|   Microchip Technology Inc.
|   PolarFire IBIS Model
[IBIS ver]   5.0
[File name]   polarfire_hsio_se.ibs
[File Rev]   2.2
[Date]   Wed Nov 22 2023
[Source] Simulated Models ONLY.
   All data is based on Spice simulation. All performed at Microchip Technology Inc.
[Notes]   This IBIS file is for HSIO single ended standards.
   Please refer to polarfire_hsio_diff.ibs for HSIO differential Standards Configurations,
   and refer to polarfire_gpio_se.ibs and polarfire_gpio_diff.ibs for GPIO Configurations.
   The package parasitics of various package types are given.
   Uncomment the appropriate package before simulations.
   Revision History
   Rev 2.2: 22-Nov-2023
   - Added mixed mode receiver support:
   - Input buffers: LVCMOS12_135_ODT-OFF,LVCMOS12_135_ODT-120,LVCMOS12_135_ODT-240,
   HSTL12_18_ODT-OFF,HSTL12_15_ODT-OFF,HSTL12_135_ODT-OFF,
   HSTL135_18_ODT-OFF,HSTL135_15_ODT-OFF,HSTL15_18_ODT-OFF,
   HSUL12_18_ODT-OFF,HSUL12_18_ODT-60,HSUL12_18_ODT-120,HSUL12_18_ODT-240,
   HSUL12_15_ODT-OFF,HSUL12_15_ODT-60,HSUL12_15_ODT-120,HSUL12_15_ODT-240,
   HSUL12_135_ODT-OFF,HSUL12_135_ODT-60,HSUL12_135_ODT-120,HSUL12_135_ODT-240,
   POD12_18_ODT-OFF,POD12_15_ODT-OFF,POD12_135_ODT-OFF,SSTL135_18_ODT-OFF,
   SSTL135_15_ODT-OFF,SSTL15_18_ODT-OFF
   Rev 2.1: 14-Sep-2022
   - Added MPF050 device with RLC package data in [Package] section
   - Component name change to PolarFire
   - Added LPDDR4 LVSTL11 I/O standard
   - Added RLC package type of FCG784N for MPF300T/TS device
   - Update RLC values of 200T-FCVG484 device package data
[Disclaimer] This information is for board design considerations.
   Simulation based V/I curves contained in this model file are
   considered preliminary until verified against bench
   measurements. Maximum currents may vary from part to part but
   should not exceed maximum I/V curves provided in this model file.
[Copyright]  (c) 2023, Microchip Technology Inc., All Rights Reserved.
| ADDITIONAL NOTES
| Warnings for ISSO Pullup, Pulldown currents being non-zero maybe ignored.
| The naming conventions used in the signal_name/model_name are as follows:
| SLEW-#  - Slew setting,OFF or ON represented by #
| HYST-#  - Hysteresis setting,OFF or ON represented by #
| #mA   - Driver current strength, value represented by #
| #ohm   - Driver impedance mode, value represented by #
| ODT-#   - Series on-die termination, impedance value represented by #
| C1   - Refers to Class-I driver models
| C2   - Refers to Class-II driver models
| #_I   - Refers to input models ,  model name represented by #
| #_O   - Refers to output models , model name represented by #
| IBIS MODEL CHECKLIST
| Microchip Technology Inc. is dedicated to releasing quality IBIS models to customers.
| The following items have been
| verified for this IBIS model before release:
| 1)  Checked IBIS model by the golden parser ibischk5 [Complete]
| 2)  Ensured no errors reported by golden parser
|   for the IBIS model [Complete]
| 3)  Defined Vinl and Vinh for receivers [Complete]
| 4)  Defined Standard Load and Vmeas values for drivers [Complete]
| 5)  Defined overshoots for drivers and receivers [NA]
| 6)  Validated Ramp Values[]
| 7)  Defined V-T Tables for all output drivers [Complete]
| 8)  Validated [Diff Pins] [NA]
| 9)  Verified Package Parasitics [Complete]
| 10) Defined Standard Load Parameters and Specifications
|   for waveforms [Complete]
| 11) Defined and Validate Pin mappings [Complete]
| 12) Verified C_comp_pullup and C_comp_pulldown Values []
| 13) Visually Inspected I-V Curves and V-T Tables  [Complete]
| 14) Presented Typ/Min/Max Values in the correct order for
|   all tables and parameters [Complete]
| 15) Simulated all output models with standard load and
|   switching through Vmeas [Complete]
| 16) Simulated all receiver models  [Complete]
| 17) Validated Models selectors. [NA]
| 18) Visually inspected Spice and IBIS correlation for
|   a) Typical VT Curves [Complete]
|   b) Minimum VT Curves [Complete]
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[Component]   PolarFire
[Manufacturer]   Microchip Technology Inc.
[Package]
|   typ   min   max
|MPF050T/TL/TLS/TS
|R_pkg   0.424   NA   NA   | MPF050T/TL/TLS/TS-FCSG325
|L_pkg   2.847nH   NA   NA   | MPF050T/TL/TLS/TS-FCSG325
|C_pkg   1.075pF   NA   NA   | MPF050T/TL/TLS/TS-FCSG325
|R_pkg   0.726   NA   NA   | MPF050T/TL/TLS/TS-FCVG484
|L_pkg   5.270nH   NA   NA   | MPF050T/TL/TLS/TS-FCVG484
|C_pkg   1.827pF   NA   NA   | MPF050T/TL/TLS/TS-FCVG484
|MPF100T/TL/TLS/TS
|R_pkg   0.300925   NA   NA   | MPF100T/TL/TLS/TS-FCSG325
|L_pkg   2.47653nH   NA   NA   | MPF100T/TL/TLS/TS-FCSG325
|C_pkg   1.00755pF   NA   NA   | MPF100T/TL/TLS/TS-FCSG325
|R_pkg   0.873007   NA   NA   | MPF100T/TL/TLS/TS-FCG484
|L_pkg   5.7244nH   NA   NA   | MPF100T/TL/TLS/TS-FCG484
|C_pkg   2.04208pF   NA   NA   | MPF100T/TL/TLS/TS-FCG484
|R_pkg   0.61   NA   NA   | MPF100T/TL/TLS/TS-FCVG484
|L_pkg   4.49536nH   NA   NA   | MPF100T/TL/TLS/TS-FCVG484
|C_pkg   1.77743pF   NA   NA   | MPF100T/TL/TLS/TS-FCVG484
|MPF200T/TL/TLS/TS
|R_pkg   0.570552   NA   NA   | MPF200T/TL/TLS/TS-FCSG325
|L_pkg   4.57321nH   NA   NA   | MPF200T/TL/TLS/TS-FCSG325
|C_pkg   1.39793pF   NA   NA   | MPF200T/TL/TLS/TS-FCSG325
|R_pkg   0.813737   NA   NA   | MPF200T/TL/TLS/TS-FCG484
|L_pkg   5.39433nH   NA   NA   | MPF200T/TL/TLS/TS-FCG484
|C_pkg   1.90867pF   NA   NA   | MPF200T/TL/TLS/TS-FCG484
|R_pkg   0.592554   NA   NA   | MPF200T/TL/TLS/TS-FCVG484
|L_pkg   4.00867nH   NA   NA   | MPF200T/TL/TLS/TS-FCVG484
|C_pkg   1.56354pF   NA   NA   | MPF200T/TL/TLS/TS-FCVG484
|R_pkg   0.39999   NA   NA   | MPF200T/TL/TLS/TS-FCSG536
|L_pkg   3.20603nH   NA   NA   | MPF200T/TL/TLS/TS-FCSG536
|C_pkg   1.22995pF   NA   NA   | MPF200T/TL/TLS/TS-FCSG536
|R_pkg   1.32073   NA   NA   | MPF200T/TL/TLS/TS-FCG784
|L_pkg   8.15293nH   NA   NA   | MPF200T/TL/TLS/TS-FCG784
|C_pkg   2.72193pF   NA   NA   | MPF200T/TL/TLS/TS-FCG784
|MPF300T/TL/TLS/TS
|R_pkg   0.713491   NA   NA   | MPF300T/TL/TLS/TS-FCG484
|L_pkg   4.77635nH   NA   NA   | MPF300T/TL/TLS/TS-FCG484
|C_pkg   1.82577pF   NA   NA   | MPF300T/TL/TLS/TS-FCG484
|R_pkg   0.493927   NA   NA   | MPF300T/TL/TLS/TS-FCVG484
|L_pkg   3.29806nH   NA   NA   | MPF300T/TL/TLS/TS-FCVG484
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R_pkg   1.65645   NA   NA   | MPF300T/TL/TLS/TS-FCG1152
L_pkg   9.92288nH   NA   NA   | MPF300T/TL/TLS/TS-FCG1152
C_pkg   3.06321pF   NA   NA   | MPF300T/TL/TLS/TS-FCG1152
|MPF500T/TL/TLS/TS
|R_pkg   0.914871   NA   NA   | MPF500T/TL/TLS/TS-FCG784
|L_pkg   5.88658nH   NA   NA   | MPF500T/TL/TLS/TS-FCG784
|C_pkg   2.0993pF   NA   NA   | MPF500T/TL/TLS/TS-FCG784
|R_pkg   1.46382   NA   NA   | MPF500T/TL/TLS/TS-FCG1152
|L_pkg   9.31721nH   NA   NA   | MPF500T/TL/TLS/TS-FCG1152
|C_pkg   2.98723pF   NA   NA   | MPF500T/TL/TLS/TS-FCG1152
| End Header
| The PIN numbers given below are examples. They do not correspond to
| device pin numbers.
[Pin]   signal_name   model_name   R_pin   L_pin   C_pin
1   LVCMOS18_8mA_SLEW-OFF_O   LVCMOS18_8mA_SLEW-OFF_HSIO_O
2   LVCMOS18_2mA_SLEW-OFF_O   LVCMOS18_2mA_SLEW-OFF_HSIO_O
3   LVCMOS18_4mA_SLEW-OFF_O   LVCMOS18_4mA_SLEW-OFF_HSIO_O
4   LVCMOS18_6mA_SLEW-OFF_O   LVCMOS18_6mA_SLEW-OFF_HSIO_O
5   LVCMOS18_10mA_SLEW-OFF_O   LVCMOS18_10mA_SLEW-OFF_HSIO_O
6   LVCMOS18_12mA_SLEW-OFF_O   LVCMOS18_12mA_SLEW-OFF_HSIO_O
7   LVCMOS15_8mA_SLEW-OFF_O   LVCMOS15_8mA_SLEW-OFF_HSIO_O
8   LVCMOS15_2mA_SLEW-OFF_O   LVCMOS15_2mA_SLEW-OFF_HSIO_O
9   LVCMOS15_4mA_SLEW-OFF_O   LVCMOS15_4mA_SLEW-OFF_HSIO_O
10   LVCMOS15_6mA_SLEW-OFF_O   LVCMOS15_6mA_SLEW-OFF_HSIO_O
11   LVCMOS15_10mA_SLEW-OFF_O   LVCMOS15_10mA_SLEW-OFF_HSIO_O
12   LVCMOS12_8mA_SLEW-OFF_O   LVCMOS12_8mA_SLEW-OFF_HSIO_O
13   LVCMOS12_2mA_SLEW-OFF_O   LVCMOS12_2mA_SLEW-OFF_HSIO_O
14   LVCMOS12_4mA_SLEW-OFF_O   LVCMOS12_4mA_SLEW-OFF_HSIO_O
15   LVCMOS12_6mA_SLEW-OFF_O   LVCMOS12_6mA_SLEW-OFF_HSIO_O
16   LVCMOS12_10mA_SLEW-OFF_O   LVCMOS12_10mA_SLEW-OFF_HSIO_O
17   SSTL18_C1_60ohm_SLEW-OFF_O   SSTL18_C1_60ohm_SLEW-OFF_HSIO_O
18   SSTL18_C1_80ohm_SLEW-OFF_O   SSTL18_C1_80ohm_SLEW-OFF_HSIO_O
19   SSTL18_C1_48ohm_SLEW-OFF_O   SSTL18_C1_48ohm_SLEW-OFF_HSIO_O
20   SSTL18_C1_40ohm_SLEW-OFF_O   SSTL18_C1_40ohm_SLEW-OFF_HSIO_O
21   SSTL18_C2_40ohm_SLEW-OFF_O   SSTL18_C2_40ohm_SLEW-OFF_HSIO_O
22   SSTL18_C2_48ohm_SLEW-OFF_O   SSTL18_C2_48ohm_SLEW-OFF_HSIO_O
23   SSTL18_C2_34ohm_SLEW-OFF_O   SSTL18_C2_34ohm_SLEW-OFF_HSIO_O
24   SSTL18_C2_30ohm_SLEW-OFF_O   SSTL18_C2_30ohm_SLEW-OFF_HSIO_O
25   SSTL15_C1_40ohm_SLEW-OFF_O   SSTL15_C1_40ohm_SLEW-OFF_HSIO_O
26   SSTL15_C1_48ohm_SLEW-OFF_O   SSTL15_C1_48ohm_SLEW-OFF_HSIO_O
27   SSTL15_C2_34ohm_SLEW-OFF_O   SSTL15_C2_34ohm_SLEW-OFF_HSIO_O
28   SSTL15_C2_30ohm_SLEW-OFF_O   SSTL15_C2_30ohm_SLEW-OFF_HSIO_O
29   SSTL15_C2_27ohm_SLEW-OFF_O   SSTL15_C2_27ohm_SLEW-OFF_HSIO_O
30   SSTL135_C1_40ohm_SLEW-OFF_O   SSTL135_C1_40ohm_SLEW-OFF_HSIO_O
31   SSTL135_C1_48ohm_SLEW-OFF_O   SSTL135_C1_48ohm_SLEW-OFF_HSIO_O
32   SSTL135_C2_34ohm_SLEW-OFF_O   SSTL135_C2_34ohm_SLEW-OFF_HSIO_O
33   SSTL135_C2_30ohm_SLEW-OFF_O   SSTL135_C2_30ohm_SLEW-OFF_HSIO_O
34   SSTL135_C2_27ohm_SLEW-OFF_O   SSTL135_C2_27ohm_SLEW-OFF_HSIO_O
35   HSUL18_C1_55ohm_SLEW-OFF_O   HSUL18_C1_55ohm_SLEW-OFF_HSIO_O
36   HSUL18_C1_60ohm_SLEW-OFF_O   HSUL18_C1_60ohm_SLEW-OFF_HSIO_O
37   HSUL18_C1_40ohm_SLEW-OFF_O   HSUL18_C1_40ohm_SLEW-OFF_HSIO_O
38   HSUL18_C1_34ohm_SLEW-OFF_O   HSUL18_C1_34ohm_SLEW-OFF_HSIO_O
39   HSUL18_C2_25ohm_SLEW-OFF_O   HSUL18_C2_25ohm_SLEW-OFF_HSIO_O
40   HSUL18_C2_30ohm_SLEW-OFF_O   HSUL18_C2_30ohm_SLEW-OFF_HSIO_O
41   HSUL18_C2_27ohm_SLEW-OFF_O   HSUL18_C2_27ohm_SLEW-OFF_HSIO_O
42   HSUL18_C2_22ohm_SLEW-OFF_O   HSUL18_C2_22ohm_SLEW-OFF_HSIO_O
43   HSTL15_C1_50ohm_SLEW-OFF_O   HSTL15_C1_50ohm_SLEW-OFF_HSIO_O
44   HSTL15_C1_60ohm_SLEW-OFF_O   HSTL15_C1_60ohm_SLEW-OFF_HSIO_O
45   HSTL15_C1_40ohm_SLEW-OFF_O   HSTL15_C1_40ohm_SLEW-OFF_HSIO_O
46   HSTL15_C1_34ohm_SLEW-OFF_O   HSTL15_C1_34ohm_SLEW-OFF_HSIO_O
47   HSTL15_C2_25ohm_SLEW-OFF_O   HSTL15_C2_25ohm_SLEW-OFF_HSIO_O
48   HSTL15_C2_30ohm_SLEW-OFF_O   HSTL15_C2_30ohm_SLEW-OFF_HSIO_O
49   HSTL15_C2_27ohm_SLEW-OFF_O   HSTL15_C2_27ohm_SLEW-OFF_HSIO_O
50   HSTL15_C2_22ohm_SLEW-OFF_O   HSTL15_C2_22ohm_SLEW-OFF_HSIO_O
51   HSTL135_C1_50ohm_SLEW-OFF_O   HSTL135_C1_50ohm_SLEW-OFF_HSIO_O
52   HSTL135_C1_60ohm_SLEW-OFF_O   HSTL135_C1_60ohm_SLEW-OFF_HSIO_O
53   HSTL135_C1_40ohm_SLEW-OFF_O   HSTL135_C1_40ohm_SLEW-OFF_HSIO_O
54   HSTL135_C1_34ohm_SLEW-OFF_O   HSTL135_C1_34ohm_SLEW-OFF_HSIO_O
55   HSTL135_C2_25ohm_SLEW-OFF_O   HSTL135_C2_25ohm_SLEW-OFF_HSIO_O
56   HSTL135_C2_30ohm_SLEW-OFF_O   HSTL135_C2_30ohm_SLEW-OFF_HSIO_O
57   HSTL135_C2_27ohm_SLEW-OFF_O   HSTL135_C2_27ohm_SLEW-OFF_HSIO_O
58   HSTL135_C2_22ohm_SLEW-OFF_O   HSTL135_C2_22ohm_SLEW-OFF_HSIO_O
59   HSUL12_40ohm_SLEW-OFF_O   HSUL12_40ohm_SLEW-OFF_HSIO_O
60   HSUL12_120ohm_SLEW-OFF_O   HSUL12_120ohm_SLEW-OFF_HSIO_O
61   HSUL12_80ohm_SLEW-OFF_O   HSUL12_80ohm_SLEW-OFF_HSIO_O
62   HSUL12_60ohm_SLEW-OFF_O   HSUL12_60ohm_SLEW-OFF_HSIO_O
63   HSUL12_48ohm_SLEW-OFF_O   HSUL12_48ohm_SLEW-OFF_HSIO_O
64   HSUL12_34ohm_SLEW-OFF_O   HSUL12_34ohm_SLEW-OFF_HSIO_O
65   POD12_C1_48ohm_SLEW-OFF_O   POD12_C1_48ohm_SLEW-OFF_HSIO_O
66   POD12_C1_60ohm_SLEW-OFF_O   POD12_C1_60ohm_SLEW-OFF_HSIO_O
67   POD12_C1_40ohm_SLEW-OFF_O   POD12_C1_40ohm_SLEW-OFF_HSIO_O
68   POD12_C2_34ohm_SLEW-OFF_O   POD12_C2_34ohm_SLEW-OFF_HSIO_O
69   POD12_C2_30ohm_SLEW-OFF_O   POD12_C2_30ohm_SLEW-OFF_HSIO_O
70   POD12_C2_27ohm_SLEW-OFF_O   POD12_C2_27ohm_SLEW-OFF_HSIO_O
71   HSTL12_C1_50ohm_SLEW-OFF_O   HSTL12_C1_50ohm_SLEW-OFF_HSIO_O
72   HSTL12_C2_25ohm_SLEW-OFF_O   HSTL12_C2_25ohm_SLEW-OFF_HSIO_O
73   LVCMOS18_ODT-OFF_HYST-ON_I   LVCMOS18_ODT-OFF_HYST-ON_HSIO_I
74   LVCMOS18_ODT-OFF_HYST-OFF_I   LVCMOS18_ODT-OFF_HYST-OFF_HSIO_I
75   LVCMOS18_ODT-120_HYST-ON_I   LVCMOS18_ODT-120_HYST-ON_HSIO_I
76   LVCMOS18_ODT-240_HYST-ON_I   LVCMOS18_ODT-240_HYST-ON_HSIO_I
77   LVCMOS18_ODT-120_HYST-OFF_I   LVCMOS18_ODT-120_HYST-OFF_HSIO_I
78   LVCMOS18_ODT-240_HYST-OFF_I   LVCMOS18_ODT-240_HYST-OFF_HSIO_I
79   LVCMOS15_18_ODT-OFF_HYST-ON_I   LVCMOS15_18_ODT-OFF_HYST-ON_HSIO_I
80   LVCMOS15_18_ODT-OFF_HYST-OFF_I   LVCMOS15_18_ODT-OFF_HYST-OFF_HSIO_I
81   LVCMOS15_18_ODT-120_HYST-ON_I   LVCMOS15_18_ODT-120_HYST-ON_HSIO_I
82   LVCMOS15_18_ODT-240_HYST-ON_I   LVCMOS15_18_ODT-240_HYST-ON_HSIO_I
83   LVCMOS15_18_ODT-120_HYST-OFF_I   LVCMOS15_18_ODT-120_HYST-OFF_HSIO_I
84   LVCMOS15_18_ODT-240_HYST-OFF_I   LVCMOS15_18_ODT-240_HYST-OFF_HSIO_I
85   LVCMOS15_ODT-OFF_HYST-ON_I   LVCMOS15_ODT-OFF_HYST-ON_HSIO_I
86   LVCMOS15_ODT-OFF_HYST-OFF_I   LVCMOS15_ODT-OFF_HYST-OFF_HSIO_I
87   LVCMOS15_ODT-120_HYST-ON_I   LVCMOS15_ODT-120_HYST-ON_HSIO_I
88   LVCMOS15_ODT-240_HYST-ON_I   LVCMOS15_ODT-240_HYST-ON_HSIO_I
89   LVCMOS15_ODT-120_HYST-OFF_I   LVCMOS15_ODT-120_HYST-OFF_HSIO_I
90   LVCMOS15_ODT-240_HYST-OFF_I   LVCMOS15_ODT-240_HYST-OFF_HSIO_I
91   LVCMOS12_18_ODT-OFF_HYST-OFF_I   LVCMOS12_18_ODT-OFF_HYST-OFF_HSIO_I
92   LVCMOS12_15_ODT-OFF_HYST-OFF_I   LVCMOS12_15_ODT-OFF_HYST-OFF_HSIO_I
93   LVCMOS12_18_ODT-120_HYST-OFF_I   LVCMOS12_18_ODT-120_HYST-OFF_HSIO_I
94   LVCMOS12_15_ODT-120_HYST-OFF_I   LVCMOS12_15_ODT-120_HYST-OFF_HSIO_I
95   LVCMOS12_18_ODT-240_HYST-OFF_I   LVCMOS12_18_ODT-240_HYST-OFF_HSIO_I
96   LVCMOS12_15_ODT-240_HYST-OFF_I   LVCMOS12_15_ODT-240_HYST-OFF_HSIO_I
97   LVCMOS12_ODT-OFF_HYST-OFF_I   LVCMOS12_ODT-OFF_HYST-OFF_HSIO_I
98   LVCMOS12_ODT-120_HYST-OFF_I   LVCMOS12_ODT-120_HYST-OFF_HSIO_I
99   LVCMOS12_ODT-240_HYST-OFF_I   LVCMOS12_ODT-240_HYST-OFF_HSIO_I
100   SSTL18_ODT-OFF_HYST-OFF_I   SSTL18_ODT-OFF_HYST-OFF_HSIO_I
101   SSTL18_ODT-50_HYST-OFF_I   SSTL18_ODT-50_HYST-OFF_HSIO_I
102   SSTL18_ODT-150_HYST-OFF_I   SSTL18_ODT-150_HYST-OFF_HSIO_I
103   SSTL18_ODT-75_HYST-OFF_I   SSTL18_ODT-75_HYST-OFF_HSIO_I
104   SSTL15_ODT-OFF_HYST-OFF_I   SSTL15_ODT-OFF_HYST-OFF_HSIO_I
105   SSTL15_ODT-60_HYST-OFF_I   SSTL15_ODT-60_HYST-OFF_HSIO_I
106   SSTL15_ODT-120_HYST-OFF_I   SSTL15_ODT-120_HYST-OFF_HSIO_I
107   SSTL15_ODT-40_HYST-OFF_I   SSTL15_ODT-40_HYST-OFF_HSIO_I
108   SSTL15_ODT-30_HYST-OFF_I   SSTL15_ODT-30_HYST-OFF_HSIO_I
109   SSTL15_ODT-20_HYST-OFF_I   SSTL15_ODT-20_HYST-OFF_HSIO_I
110   SSTL135_ODT-OFF_HYST-OFF_I   SSTL135_ODT-OFF_HYST-OFF_HSIO_I
111   SSTL135_ODT-60_HYST-OFF_I   SSTL135_ODT-60_HYST-OFF_HSIO_I
112   SSTL135_ODT-120_HYST-OFF_I   SSTL135_ODT-120_HYST-OFF_HSIO_I
113   SSTL135_ODT-40_HYST-OFF_I   SSTL135_ODT-40_HYST-OFF_HSIO_I
114   SSTL135_ODT-30_HYST-OFF_I   SSTL135_ODT-30_HYST-OFF_HSIO_I
115   SSTL135_ODT-20_HYST-OFF_I   SSTL135_ODT-20_HYST-OFF_HSIO_I
116   HSUL18_ODT-OFF_HYST-OFF_I   HSUL18_ODT-OFF_HYST-OFF_HSIO_I
117   HSUL18_ODT-50_HYST-OFF_I   HSUL18_ODT-50_HYST-OFF_HSIO_I
118   HSTL15_ODT-OFF_HYST-OFF_I   HSTL15_ODT-OFF_HYST-OFF_HSIO_I
119   HSTL15_ODT-50_HYST-OFF_I   HSTL15_ODT-50_HYST-OFF_HSIO_I
120   HSTL135_ODT-OFF_HYST-OFF_I   HSTL135_ODT-OFF_HYST-OFF_HSIO_I
121   HSTL135_ODT-50_HYST-OFF_I   HSTL135_ODT-50_HYST-OFF_HSIO_I
122   HSUL12_ODT-OFF_HYST-OFF_I   HSUL12_ODT-OFF_HYST-OFF_HSIO_I
123   HSUL12_ODT-60_HYST-OFF_I   HSUL12_ODT-60_HYST-OFF_HSIO_I
124   HSUL12_ODT-240_HYST-OFF_I   HSUL12_ODT-240_HYST-OFF_HSIO_I
125   HSUL12_ODT-120_HYST-OFF_I   HSUL12_ODT-120_HYST-OFF_HSIO_I
126   POD12_ODT-OFF_HYST-OFF_I   POD12_ODT-OFF_HYST-OFF_HSIO_I
127   POD12_ODT-60_HYST-OFF_I   POD12_ODT-60_HYST-OFF_HSIO_I
128   POD12_ODT-240_HYST-OFF_I   POD12_ODT-240_HYST-OFF_HSIO_I
129   POD12_ODT-120_HYST-OFF_I   POD12_ODT-120_HYST-OFF_HSIO_I
130   POD12_ODT-80_HYST-OFF_I   POD12_ODT-80_HYST-OFF_HSIO_I
131   POD12_ODT-48_HYST-OFF_I   POD12_ODT-48_HYST-OFF_HSIO_I
132   POD12_ODT-40_HYST-OFF_I   POD12_ODT-40_HYST-OFF_HSIO_I
133   POD12_ODT-34_HYST-OFF_I   POD12_ODT-34_HYST-OFF_HSIO_I
134   HSTL12_ODT-OFF_HYST-OFF_I   HSTL12_ODT-OFF_HYST-OFF_HSIO_I
135   HSTL12_ODT-50_HYST-OFF_I   HSTL12_ODT-50_HYST-OFF_HSIO_I
136   LVSTL11_C1_40ohm_SLEW-OFF_O   LVSTL11_C1_40ohm_SLEW-OFF_HSIO_O
137   LVSTL11_C1_120ohm_SLEW-OFF_O   LVSTL11_C1_120ohm_SLEW-OFF_HSIO_O
138   LVSTL11_C1_80ohm_SLEW-OFF_O   LVSTL11_C1_80ohm_SLEW-OFF_HSIO_O
139   LVSTL11_C1_60ohm_SLEW-OFF_O   LVSTL11_C1_60ohm_SLEW-OFF_HSIO_O
140   LVSTL11_C1_48ohm_SLEW-OFF_O   LVSTL11_C1_48ohm_SLEW-OFF_HSIO_O
141   LVSTL11_C1_34ohm_SLEW-OFF_O   LVSTL11_C1_34ohm_SLEW-OFF_HSIO_O
142   LVSTL11_ODT-OFF_HYST-OFF_I   LVSTL11_ODT-OFF_HYST-OFF_HSIO_I
143   LVSTL11_ODT-60_HYST-OFF_I   LVSTL11_ODT-60_HYST-OFF_HSIO_I
144   LVSTL11_ODT-120_HYST-OFF_I   LVSTL11_ODT-120_HYST-OFF_HSIO_I
145   LVSTL11_ODT-80_HYST-OFF_I   LVSTL11_ODT-80_HYST-OFF_HSIO_I
146   LVSTL11_ODT-48_HYST-OFF_I   LVSTL11_ODT-48_HYST-OFF_HSIO_I
147   LVSTL11_ODT-40_HYST-OFF_I   LVSTL11_ODT-40_HYST-OFF_HSIO_I
148   LVCMOS12_135_ODT-OFF_HYST-OFF_I   LVCMOS12_135_ODT-OFF_HYST-OFF_HSIO_I
149   LVCMOS12_135_ODT-120_HYST-OFF_I   LVCMOS12_135_ODT-120_HYST-OFF_HSIO_I
150   LVCMOS12_135_ODT-240_HYST-OFF_I   LVCMOS12_135_ODT-240_HYST-OFF_HSIO_I
151   HSTL12_18_ODT-OFF_HYST-OFF_I   HSTL12_18_ODT-OFF_HYST-OFF_HSIO_I
152   HSTL12_15_ODT-OFF_HYST-OFF_I   HSTL12_15_ODT-OFF_HYST-OFF_HSIO_I
153   HSTL12_135_ODT-OFF_HYST-OFF_I   HSTL12_135_ODT-OFF_HYST-OFF_HSIO_I
154   HSTL135_18_ODT-OFF_HYST-OFF_I   HSTL135_18_ODT-OFF_HYST-OFF_HSIO_I
155   HSTL135_15_ODT-OFF_HYST-OFF_I   HSTL135_15_ODT-OFF_HYST-OFF_HSIO_I
156   HSTL15_18_ODT-OFF_HYST-OFF_I   HSTL15_18_ODT-OFF_HYST-OFF_HSIO_I
157   HSUL12_18_ODT-OFF_HYST-OFF_I   HSUL12_18_ODT-OFF_HYST-OFF_HSIO_I
158   HSUL12_15_ODT-OFF_HYST-OFF_I   HSUL12_15_ODT-OFF_HYST-OFF_HSIO_I
159   HSUL12_135_ODT-OFF_HYST-OFF_I   HSUL12_135_ODT-OFF_HYST-OFF_HSIO_I
160   HSUL12_18_ODT-60_HYST-OFF_I   HSUL12_18_ODT-60_HYST-OFF_HSIO_I
161   HSUL12_15_ODT-60_HYST-OFF_I   HSUL12_15_ODT-60_HYST-OFF_HSIO_I
162   HSUL12_135_ODT-60_HYST-OFF_I   HSUL12_135_ODT-60_HYST-OFF_HSIO_I
163   HSUL12_18_ODT-240_HYST-OFF_I   HSUL12_18_ODT-240_HYST-OFF_HSIO_I
164   HSUL12_15_ODT-240_HYST-OFF_I   HSUL12_15_ODT-240_HYST-OFF_HSIO_I
165   HSUL12_135_ODT-240_HYST-OFF_I   HSUL12_135_ODT-240_HYST-OFF_HSIO_I
166   HSUL12_18_ODT-120_HYST-OFF_I   HSUL12_18_ODT-120_HYST-OFF_HSIO_I
167   HSUL12_15_ODT-120_HYST-OFF_I   HSUL12_15_ODT-120_HYST-OFF_HSIO_I
168   HSUL12_135_ODT-120_HYST-OFF_I   HSUL12_135_ODT-120_HYST-OFF_HSIO_I
169   POD12_18_ODT-OFF_HYST-OFF_I   POD12_18_ODT-OFF_HYST-OFF_HSIO_I
170   POD12_15_ODT-OFF_HYST-OFF_I   POD12_15_ODT-OFF_HYST-OFF_HSIO_I
171   POD12_135_ODT-OFF_HYST-OFF_I   POD12_135_ODT-OFF_HYST-OFF_HSIO_I
172   SSTL135_18_ODT-OFF_HYST-OFF_I   SSTL135_18_ODT-OFF_HYST-OFF_HSIO_I
173   SSTL135_15_ODT-OFF_HYST-OFF_I   SSTL135_15_ODT-OFF_HYST-OFF_HSIO_I
174   SSTL15_18_ODT-OFF_HYST-OFF_I   SSTL15_18_ODT-OFF_HYST-OFF_HSIO_I
175   VDDI   POWER
176   VSS   GND
[Pin Mapping]   pulldown_ref   pullup_ref   gnd_clamp_ref   power_clamp_ref   ext_ref
1   VSS   VDDI   VSS   VDDI
2   VSS   VDDI   VSS   VDDI
3   VSS   VDDI   VSS   VDDI
4   VSS   VDDI   VSS   VDDI
5   VSS   VDDI   VSS   VDDI
6   VSS   VDDI   VSS   VDDI
7   VSS   VDDI   VSS   VDDI
8   VSS   VDDI   VSS   VDDI
9   VSS   VDDI   VSS   VDDI
10   VSS   VDDI   VSS   VDDI
11   VSS   VDDI   VSS   VDDI
12   VSS   VDDI   VSS   VDDI
13   VSS   VDDI   VSS   VDDI
14   VSS   VDDI   VSS   VDDI
15   VSS   VDDI   VSS   VDDI
16   VSS   VDDI   VSS   VDDI
17   VSS   VDDI   VSS   VDDI
18   VSS   VDDI   VSS   VDDI
19   VSS   VDDI   VSS   VDDI
20   VSS   VDDI   VSS   VDDI
21   VSS   VDDI   VSS   VDDI
22   VSS   VDDI   VSS   VDDI
23   VSS   VDDI   VSS   VDDI
24   VSS   VDDI   VSS   VDDI
25   VSS   VDDI   VSS   VDDI
26   VSS   VDDI   VSS   VDDI
27   VSS   VDDI   VSS   VDDI
28   VSS   VDDI   VSS   VDDI
29   VSS   VDDI   VSS   VDDI
30   VSS   VDDI   VSS   VDDI
31   VSS   VDDI   VSS   VDDI
32   VSS   VDDI   VSS   VDDI
33   VSS   VDDI   VSS   VDDI
34   VSS   VDDI   VSS   VDDI
35   VSS   VDDI   VSS   VDDI
36   VSS   VDDI   VSS   VDDI
37   VSS   VDDI   VSS   VDDI
38   VSS   VDDI   VSS   VDDI
39   VSS   VDDI   VSS   VDDI
40   VSS   VDDI   VSS   VDDI
41   VSS   VDDI   VSS   VDDI
42   VSS   VDDI   VSS   VDDI
43   VSS   VDDI   VSS   VDDI
44   VSS   VDDI   VSS   VDDI
45   VSS   VDDI   VSS   VDDI
46   VSS   VDDI   VSS   VDDI
47   VSS   VDDI   VSS   VDDI
48   VSS   VDDI   VSS   VDDI
49   VSS   VDDI   VSS   VDDI
50   VSS   VDDI   VSS   VDDI
51   VSS   VDDI   VSS   VDDI
52   VSS   VDDI   VSS   VDDI
53   VSS   VDDI   VSS   VDDI
54   VSS   VDDI   VSS   VDDI
55   VSS   VDDI   VSS   VDDI
56   VSS   VDDI   VSS   VDDI
57   VSS   VDDI   VSS   VDDI
58   VSS   VDDI   VSS   VDDI
59   VSS   VDDI   VSS   VDDI
60   VSS   VDDI   VSS   VDDI
61   VSS   VDDI   VSS   VDDI
62   VSS   VDDI   VSS   VDDI
63   VSS   VDDI   VSS   VDDI
64   VSS   VDDI   VSS   VDDI
65   VSS   VDDI   VSS   VDDI
66   VSS   VDDI   VSS   VDDI
67   VSS   VDDI   VSS   VDDI
68   VSS   VDDI   VSS   VDDI
69   VSS   VDDI   VSS   VDDI
70   VSS   VDDI   VSS   VDDI
71   VSS   VDDI   VSS   VDDI
72   VSS   VDDI   VSS   VDDI
73   VSS   VDDI   VSS   VDDI
74   VSS   VDDI   VSS   VDDI
75   VSS   VDDI   VSS   VDDI
76   VSS   VDDI   VSS   VDDI
77   VSS   VDDI   VSS   VDDI
78   VSS   VDDI   VSS   VDDI
79   VSS   VDDI   VSS   VDDI
80   VSS   VDDI   VSS   VDDI
81   VSS   VDDI   VSS   VDDI
82   VSS   VDDI   VSS   VDDI
83   VSS   VDDI   VSS   VDDI
84   VSS   VDDI   VSS   VDDI
85   VSS   VDDI   VSS   VDDI
86   VSS   VDDI   VSS   VDDI
87   VSS   VDDI   VSS   VDDI
88   VSS   VDDI   VSS   VDDI
89   VSS   VDDI   VSS   VDDI
90   VSS   VDDI   VSS   VDDI
91   VSS   VDDI   VSS   VDDI
92   VSS   VDDI   VSS   VDDI
93   VSS   VDDI   VSS   VDDI
94   VSS   VDDI   VSS   VDDI
95   VSS   VDDI   VSS   VDDI
96   VSS   VDDI   VSS   VDDI
97   VSS   VDDI   VSS   VDDI
98   VSS   VDDI   VSS   VDDI
99   VSS   VDDI   VSS   VDDI
100   VSS   VDDI   VSS   VDDI
101   VSS   VDDI   VSS   VDDI
102   VSS   VDDI   VSS   VDDI
103   VSS   VDDI   VSS   VDDI
104   VSS   VDDI   VSS   VDDI
105   VSS   VDDI   VSS   VDDI
106   VSS   VDDI   VSS   VDDI
107   VSS   VDDI   VSS   VDDI
108   VSS   VDDI   VSS   VDDI
109   VSS   VDDI   VSS   VDDI
110   VSS   VDDI   VSS   VDDI
111   VSS   VDDI   VSS   VDDI
112   VSS   VDDI   VSS   VDDI
113   VSS   VDDI   VSS   VDDI
114   VSS   VDDI   VSS   VDDI
115   VSS   VDDI   VSS   VDDI
116   VSS   VDDI   VSS   VDDI
117   VSS   VDDI   VSS   VDDI
118   VSS   VDDI   VSS   VDDI
119   VSS   VDDI   VSS   VDDI
120   VSS   VDDI   VSS   VDDI
121   VSS   VDDI   VSS   VDDI
122   VSS   VDDI   VSS   VDDI
123   VSS   VDDI   VSS   VDDI
124   VSS   VDDI   VSS   VDDI
125   VSS   VDDI   VSS   VDDI
126   VSS   VDDI   VSS   VDDI
127   VSS   VDDI   VSS   VDDI
128   VSS   VDDI   VSS   VDDI
129   VSS   VDDI   VSS   VDDI
130   VSS   VDDI   VSS   VDDI
131   VSS   VDDI   VSS   VDDI
132   VSS   VDDI   VSS   VDDI
133   VSS   VDDI   VSS   VDDI
134   VSS   VDDI   VSS   VDDI
135   VSS   VDDI   VSS   VDDI
136   VSS   VDDI   VSS   VDDI
137   VSS   VDDI   VSS   VDDI
138   VSS   VDDI   VSS   VDDI
139   VSS   VDDI   VSS   VDDI
140   VSS   VDDI   VSS   VDDI
141   VSS   VDDI   VSS   VDDI
142   VSS   VDDI   VSS   VDDI
143   VSS   VDDI   VSS   VDDI
144   VSS   VDDI   VSS   VDDI
145   VSS   VDDI   VSS   VDDI
146   VSS   VDDI   VSS   VDDI
147   VSS   VDDI   VSS   VDDI
148   VSS   VDDI   VSS   VDDI
149   VSS   VDDI   VSS   VDDI
150   VSS   VDDI   VSS   VDDI
151   VSS   VDDI   VSS   VDDI
152   VSS   VDDI   VSS   VDDI
153   VSS   VDDI   VSS   VDDI
154   VSS   VDDI   VSS   VDDI
155   VSS   VDDI   VSS   VDDI
156   VSS   VDDI   VSS   VDDI
157   VSS   VDDI   VSS   VDDI
158   VSS   VDDI   VSS   VDDI
159   VSS   VDDI   VSS   VDDI
160   VSS   VDDI   VSS   VDDI
161   VSS   VDDI   VSS   VDDI
162   VSS   VDDI   VSS   VDDI
163   VSS   VDDI   VSS   VDDI
164   VSS   VDDI   VSS   VDDI
165   VSS   VDDI   VSS   VDDI
166   VSS   VDDI   VSS   VDDI
167   VSS   VDDI   VSS   VDDI
168   VSS   VDDI   VSS   VDDI
169   VSS   VDDI   VSS   VDDI
170   VSS   VDDI   VSS   VDDI
171   VSS   VDDI   VSS   VDDI
172   VSS   VDDI   VSS   VDDI
173   VSS   VDDI   VSS   VDDI
174   VSS   VDDI   VSS   VDDI
175   NC   VDDI
176   VSS   NC
| Models and submodels in the file (174): LVCMOS18_8mA_SLEW-OFF_HSIO_O (Output), LVCMOS18_2mA_SLEW-OFF_HSIO_O (Output), LVCMOS18_4mA_SLEW-OFF_HSIO_O (Output), LVCMOS18_6mA_SLEW-OFF_HSIO_O (Output), LVCMOS18_10mA_SLEW-OFF_HSIO_O (Output), LVCMOS18_12mA_SLEW-OFF_HSIO_O (Output), LVCMOS15_8mA_SLEW-OFF_HSIO_O (Output), LVCMOS15_2mA_SLEW-OFF_HSIO_O (Output), LVCMOS15_4mA_SLEW-OFF_HSIO_O (Output), LVCMOS15_6mA_SLEW-OFF_HSIO_O (Output), LVCMOS15_10mA_SLEW-OFF_HSIO_O (Output), LVCMOS12_8mA_SLEW-OFF_HSIO_O (Output), LVCMOS12_2mA_SLEW-OFF_HSIO_O (Output), LVCMOS12_4mA_SLEW-OFF_HSIO_O (Output), LVCMOS12_6mA_SLEW-OFF_HSIO_O (Output), LVCMOS12_10mA_SLEW-OFF_HSIO_O (Output), SSTL18_C1_60ohm_SLEW-OFF_HSIO_O (Output), SSTL18_C1_80ohm_SLEW-OFF_HSIO_O (Output), SSTL18_C1_48ohm_SLEW-OFF_HSIO_O (Output), SSTL18_C1_40ohm_SLEW-OFF_HSIO_O (Output), SSTL18_C2_40ohm_SLEW-OFF_HSIO_O (Output), SSTL18_C2_48ohm_SLEW-OFF_HSIO_O (Output), SSTL18_C2_34ohm_SLEW-OFF_HSIO_O (Output), SSTL18_C2_30ohm_SLEW-OFF_HSIO_O (Output), SSTL15_C1_40ohm_SLEW-OFF_HSIO_O (Output), SSTL15_C1_48ohm_SLEW-OFF_HSIO_O (Output), SSTL15_C2_34ohm_SLEW-OFF_HSIO_O (Output), SSTL15_C2_30ohm_SLEW-OFF_HSIO_O (Output), SSTL15_C2_27ohm_SLEW-OFF_HSIO_O (Output), SSTL135_C1_40ohm_SLEW-OFF_HSIO_O (Output), SSTL135_C1_48ohm_SLEW-OFF_HSIO_O (Output), SSTL135_C2_34ohm_SLEW-OFF_HSIO_O (Output), SSTL135_C2_30ohm_SLEW-OFF_HSIO_O (Output), SSTL135_C2_27ohm_SLEW-OFF_HSIO_O (Output), HSUL18_C1_55ohm_SLEW-OFF_HSIO_O (Output), HSUL18_C1_60ohm_SLEW-OFF_HSIO_O (Output), HSUL18_C1_40ohm_SLEW-OFF_HSIO_O (Output), HSUL18_C1_34ohm_SLEW-OFF_HSIO_O (Output), HSUL18_C2_25ohm_SLEW-OFF_HSIO_O (Output), HSUL18_C2_30ohm_SLEW-OFF_HSIO_O (Output), HSUL18_C2_27ohm_SLEW-OFF_HSIO_O (Output), HSUL18_C2_22ohm_SLEW-OFF_HSIO_O (Output), HSTL15_C1_50ohm_SLEW-OFF_HSIO_O (Output), HSTL15_C1_60ohm_SLEW-OFF_HSIO_O (Output), HSTL15_C1_40ohm_SLEW-OFF_HSIO_O (Output), HSTL15_C1_34ohm_SLEW-OFF_HSIO_O (Output), HSTL15_C2_25ohm_SLEW-OFF_HSIO_O (Output), HSTL15_C2_30ohm_SLEW-OFF_HSIO_O (Output), HSTL15_C2_27ohm_SLEW-OFF_HSIO_O (Output), HSTL15_C2_22ohm_SLEW-OFF_HSIO_O (Output), HSTL135_C1_50ohm_SLEW-OFF_HSIO_O (Output), HSTL135_C1_60ohm_SLEW-OFF_HSIO_O (Output), HSTL135_C1_40ohm_SLEW-OFF_HSIO_O (Output), HSTL135_C1_34ohm_SLEW-OFF_HSIO_O (Output), HSTL135_C2_25ohm_SLEW-OFF_HSIO_O (Output), HSTL135_C2_30ohm_SLEW-OFF_HSIO_O (Output), HSTL135_C2_27ohm_SLEW-OFF_HSIO_O (Output), HSTL135_C2_22ohm_SLEW-OFF_HSIO_O (Output), HSUL12_40ohm_SLEW-OFF_HSIO_O (Output), HSUL12_120ohm_SLEW-OFF_HSIO_O (Output), HSUL12_80ohm_SLEW-OFF_HSIO_O (Output), HSUL12_60ohm_SLEW-OFF_HSIO_O (Output), HSUL12_48ohm_SLEW-OFF_HSIO_O (Output), HSUL12_34ohm_SLEW-OFF_HSIO_O (Output), POD12_C1_48ohm_SLEW-OFF_HSIO_O (Output), POD12_C1_60ohm_SLEW-OFF_HSIO_O (Output), POD12_C1_40ohm_SLEW-OFF_HSIO_O (Output), POD12_C2_34ohm_SLEW-OFF_HSIO_O (Output), POD12_C2_30ohm_SLEW-OFF_HSIO_O (Output), POD12_C2_27ohm_SLEW-OFF_HSIO_O (Output), HSTL12_C1_50ohm_SLEW-OFF_HSIO_O (Output), HSTL12_C2_25ohm_SLEW-OFF_HSIO_O (Output), LVCMOS18_ODT-OFF_HYST-ON_HSIO_I (Input), LVCMOS18_ODT-120_HYST-ON_HSIO_I (Input), LVCMOS18_ODT-240_HYST-ON_HSIO_I (Input), LVCMOS15_18_ODT-OFF_HYST-ON_HSIO_I (Input), LVCMOS15_18_ODT-120_HYST-ON_HSIO_I (Input), LVCMOS15_18_ODT-240_HYST-ON_HSIO_I (Input), LVCMOS15_ODT-OFF_HYST-ON_HSIO_I (Input), LVCMOS15_ODT-120_HYST-ON_HSIO_I (Input)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
